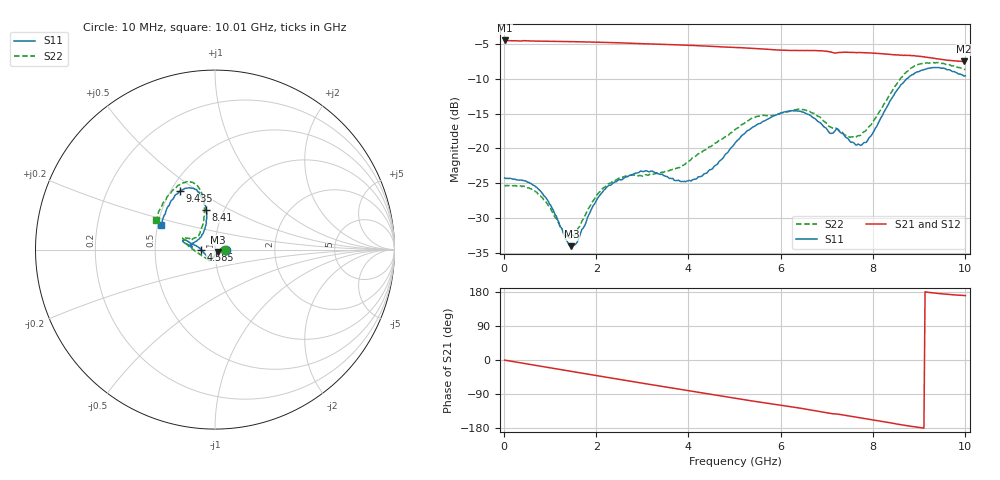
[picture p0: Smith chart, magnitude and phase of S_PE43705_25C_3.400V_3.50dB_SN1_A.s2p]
! Device ID: PE43705
! Serial: 1
! Insertion: A
! Impedance: 50 ohm
! Temp: 25C
! VDD: 3.400V
! Attenuation Step: 3.50dB
#  Hz  S  RI  R  50
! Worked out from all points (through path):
!   401 points, 10 MHz to 10.01 GHz, reference 50 ohm
!   highest |S21| = -4.53 dB at 10 MHz (marker M1); lowest = -7.5 dB at 9.985 GHz (marker M2)
!   group delay of S21, straight-line fit = 54 ps
!   lowest |S11| = -34.0 dB at 1.46 GHz (marker M3), VSWR 1.04, Z = 51.5 - j1.33 ohm
!   |S11| at or under -10 dB: start of sweep to 8.741 GHz
!   |S22| runs from -32.8 to -7.7 dB; largest |S21 - S12| = 0.0054
!   S11 on the Smith chart (normalised r, x): 10 MHz: 1.13, -0.00; 4.585 GHz: 0.86, -0.01; 8.41 GHz: 0.82, +0.39; 9.435 GHz: 0.56, +0.42; 10.01 GHz: 0.52, +0.16
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1e7  0.0615 -0.000306  0.5934 -0.00283  0.5938 -0.00282  0.0546 -0.00017
7.6e8  0.0485 0.0149  0.565 -0.1594  0.565 -0.1592  0.0446 0.0125
1.46e9  0.0152 -0.0129  0.5036 -0.2914  0.5039 -0.2914  0.016 -0.0167
1.685e9  0.0042 -0.026  0.477 -0.3295  0.4771 -0.3296  0.00504 -0.0296
2.235e9  -0.0169 -0.0505  0.3999 -0.4116  0.4002 -0.4113  -0.0188 -0.052
2.935e9  -0.0305 -0.0607  0.2827 -0.4883  0.2834 -0.4882  -0.0364 -0.0527
3.36e9  -0.0329 -0.0569  0.2061 -0.5179  0.2068 -0.5173  -0.0428 -0.0507
3.985e9  -0.0484 -0.0329  0.0877 -0.5414  0.0884 -0.5407  -0.0725 -0.0348
4.585e9  -0.0755 -0.00367  -0.0242 -0.537  -0.0234 -0.5368  -0.1089 -0.0108
5.01e9  -0.1067 0.0226  -0.0996 -0.519  -0.0993 -0.5193  -0.136 0.0104
5.435e9  -0.1392 0.0377  -0.1702 -0.4917  -0.17 -0.4925  -0.1625 0.0371
6.01e9  -0.1714 0.0539  -0.2494 -0.4399  -0.2474 -0.4403  -0.1708 0.0545
6.685e9  -0.1646 0.0339  -0.3391 -0.3704  -0.3387 -0.3702  -0.1669 0.0663
7.435e9  -0.1109 0.044  -0.408 -0.2686  -0.4073 -0.27  -0.1025 0.0704
7.71e9  -0.0818 0.0678  -0.4303 -0.2266  -0.4291 -0.2274  -0.085 0.0896
7.935e9  -0.0618 0.1037  -0.4435 -0.1909  -0.4428 -0.1934  -0.0741 0.1249
8.36e9  -0.0469 0.2095  -0.4569 -0.1197  -0.4561 -0.1215  -0.0593 0.2337
8.41e9  -0.0506 0.2224  -0.4573 -0.111  -0.4566 -0.1123  -0.061 0.2468
8.86e9  -0.0975 0.3237  -0.4604 -0.0367  -0.4573 -0.0395  -0.1112 0.3644
9.435e9  -0.197 0.3247  -0.4349 0.0353  -0.4343 0.0357  -0.2128 0.3505
9.985e9  -0.295 0.1465  -0.4133 0.0715  -0.4145 0.0711  -0.3229 0.1761
1.001e10  -0.3019 0.1368  -0.4142 0.0726  -0.4162 0.0719  -0.3304 0.1645
